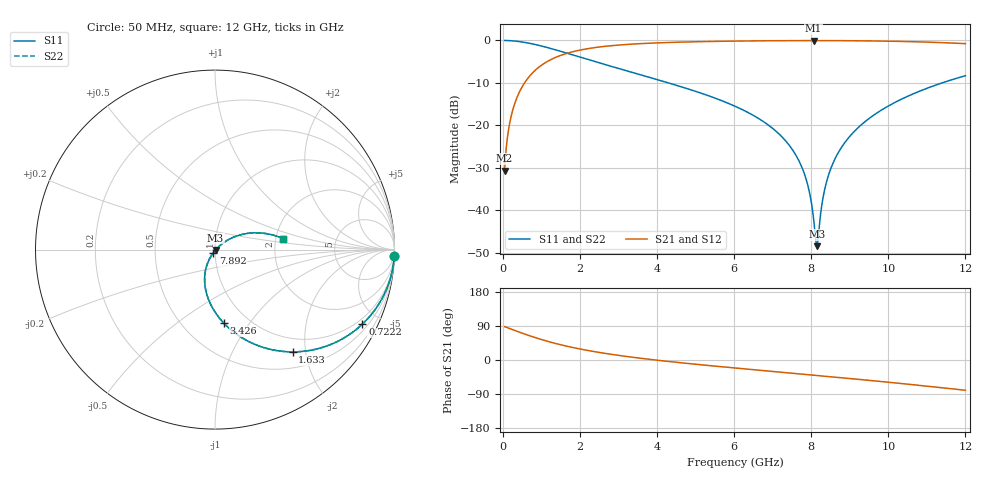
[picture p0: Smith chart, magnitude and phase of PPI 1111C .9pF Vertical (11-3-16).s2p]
# GHz S MA R 50
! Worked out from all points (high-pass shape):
!   1601 points, 50 MHz to 12 GHz, reference 50 ohm
!   highest |S21| = -0.04 dB at 8.064 GHz (marker M1); lowest = -30.7 dB at 50 MHz (marker M2)
!   |S21| within 3 dB of the highest: 1.667 GHz to end of sweep
!   lowest |S11| = -48.5 dB at 8.146 GHz (marker M3), VSWR 1.01, Z = 50.3 - j0.254 ohm
!   |S11| at or under -10 dB: 4.295 GHz to 11.4 GHz (7.103 GHz wide, 90.5 % of centre)
!   |S22| runs from -48.5 to 0.0 dB; largest |S21 - S12| = 0
!   S11 on the Smith chart (normalised r, x): 50 MHz: 1, -59; 722.2 MHz: 0.75, -4.07; 1.633 GHz: 0.75, -1.76; 3.426 GHz: 0.77, -0.76; 7.892 GHz: 0.98, -0.04; 12 GHz: 2.19, +0.32
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0.05  0.9996 -1.9  0.0293 88.1  0.0293 88.1  0.9996 -1.9
0.1620312  0.9955 -6.3  0.09457 83.7  0.09457 83.7  0.9955 -6.3
0.2815313  0.9866 -10.9  0.1629 79.1  0.1629 79.1  0.9866 -10.9
0.7221875  0.9202 -26.8  0.3909 63.2  0.3909 63.2  0.9202 -26.8
1.633375  0.7156 -52.8  0.6974 37.1  0.6974 37.1  0.7156 -52.8
2.044156  0.6291 -61.6  0.7759 28.3  0.7759 28.3  0.6291 -61.6
3.425875  0.4116 -83.3  0.9093 6.5  0.9093 6.5  0.4116 -83.3
4.038312  0.3422 -90.6  0.9373 -0.9  0.9373 -0.9  0.3422 -90.6
6.025  0.1678 -110.1  0.9827 -21.1  0.9827 -21.1  0.1678 -110.1
7.272281  0.07076 -119.9  0.9937 -32.6  0.9937 -32.6  0.07076 -119.9
7.645719  0.04115 -121.2  0.9952 -36.1  0.9952 -36.1  0.04115 -121.2
7.892188  0.02135 -118.6  0.9957 -38.4  0.9957 -38.4  0.02135 -118.6
8.019156  0.01124 -110.3  0.9958 -39.5  0.9958 -39.5  0.01124 -110.3
8.063969  0.007849 -101.7  0.9958 -40.0  0.9958 -40.0  0.007849 -101.7
8.146125  0.003763 -42.1  0.9958 -40.7  0.9958 -40.7  0.003763 -42.1
8.183469  0.004843 -2.4  0.9958 -41.1  0.9958 -41.1  0.004843 -2.4
8.288031  0.01241 29.9  0.9956 -42.1  0.9956 -42.1  0.01241 29.9
8.377656  0.01977 35.8  0.9955 -42.9  0.9955 -42.9  0.01977 35.8
8.676406  0.0453 39.2  0.9945 -45.7  0.9945 -45.7  0.0453 39.2
9.206687  0.09272 36.5  0.9909 -50.8  0.9909 -50.8  0.09272 36.5
10.01331  0.1699 29.6  0.9801 -58.8  0.9801 -58.8  0.1699 29.6
12  0.384 9.2  0.9166 -79.9  0.9166 -79.9  0.384 9.2
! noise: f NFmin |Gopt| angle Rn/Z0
0.05  0.001049  0.9714  1.708  0.008321
1.372  0.004353  0.723  11.11  0.003089
2.701  0.006904  0.6623  17.11  0.00383
4.031  0.009228  0.6324  23.16  0.004537
5.36  0.01149  0.6175  29.07  0.005264
6.682  0.01379  0.6129  34.74  0.006059
8.012  0.01623  0.616  40.2  0.006986
9.341  0.01887  0.6257  45.41  0.008105
10.67  0.02182  0.6409  50.39  0.009499
12  0.02519  0.6609  55.16  0.01129
